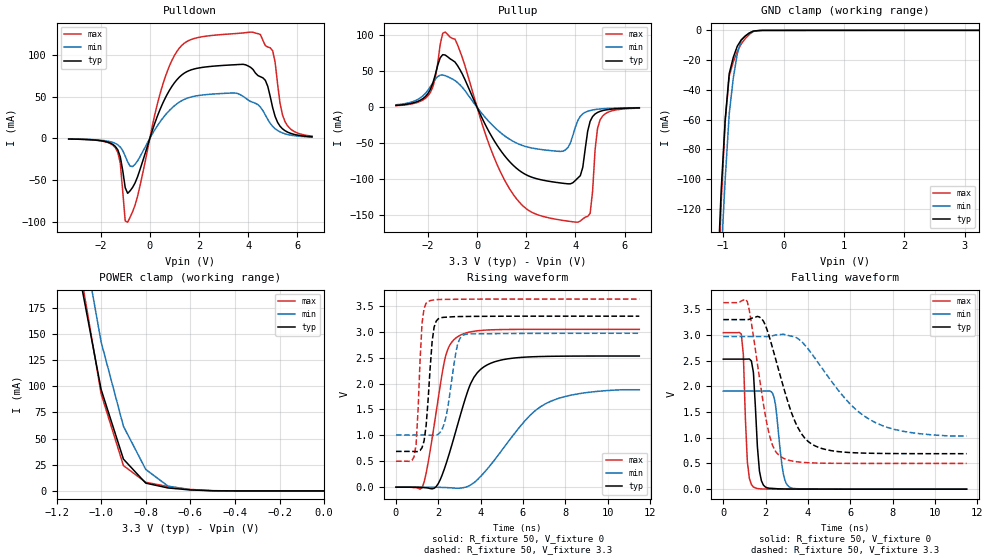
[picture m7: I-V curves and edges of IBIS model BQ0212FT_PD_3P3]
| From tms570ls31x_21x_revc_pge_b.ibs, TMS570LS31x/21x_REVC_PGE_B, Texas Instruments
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|   Model Cell BQ0212FT_PD_3P3
|BQ0212FT_PD_3P3
[Model]   BQ0212FT_PD_3P3
Model_type   I/O
Polarity   Non-Inverting
Enable   Active-Low
Vinl =  1.15
Vinh =  1.55
Cref =  15.0001pF
Rref =  101.0000M
Vref =  0V
Vmeas =  1.65
C_comp   1.2p   1.2p   1.2p
[Model Spec]
Vinl   1.15   1.02   1.28
Vinh   1.55   1.45   1.65
[Temperature Range]   25   155   -40
[Voltage Range]   3.3   2.97   3.63
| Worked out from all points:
|   slope of the pulldown table from 0 to 0.495 V, typ, clamps not added: 12.4 ohm
|   slope of the pullup table from 0 to 0.495 V, typ, clamps not added: 14.3 ohm
|   GND clamp passes 1 mA (typ) near -0.53 V on its own axis
|   POWER clamp passes 1 mA (typ) near -0.60 V on its own axis
|   rising waveform, R_fixture 50, V_fixture 0: 20-80 % time 1.15ns typ, 2.3ns min, 717ps max; typ from 0 V to 2.53 V
|   rising waveform, R_fixture 50, V_fixture 3.3: 20-80 % time 273ps typ, 440ps min, 219ps max; typ from 0.691 V to 3.3 V
|   falling waveform, R_fixture 50, V_fixture 0: 20-80 % time 219ps typ, 306ps min, 166ps max; typ from 2.53 V to 0 V
|   falling waveform, R_fixture 50, V_fixture 3.3: 20-80 % time 1.2ns typ, 2.39ns min, 725ps max; typ from 3.3 V to 0.691 V
[POWER_clamp]
|   voltage   I(typ)   I(min)   I(max)
-3.3V     3.99A      4.579A     4.788A
-1.1V     209.6mA    262.2mA    219.1mA
-1.067V   172.1mA    222.3mA    177mA
-1.033V   134.5mA    182.3mA    134.9mA
-1V       96.98mA    142.4mA    92.77mA
-900mV    30.41mA    61.81mA    24.23mA
-800mV    7.462mA    20.57mA    8.247mA
-700mV    2.848mA    4.595mA    4.228mA
-600mV    949.8uA    1.092mA    1.467mA
-500mV    155.7uA    238.9uA    226.8uA
0V        18.81uA    8.065uA    36.23uA
[Pulldown]
|   voltage   I(typ)   I(min)   I(max)
-3.3V     -649.5uA   -582.6uA   -652.5uA
-1.4V     -9.531mA   -5.889mA   -11.14mA
-1.2V     -22.05mA   -10.26mA   -29.81mA
-1V       -58.85mA   -20.91mA   -98.56mA
-900mV    -65.57mA   -28.22mA   -100.1mA
400mV     33.5mA     19.22mA    51.63mA
1.1V      70.16mA    41.36mA    104mA
4.1V      85.11mA    44.32mA    127.2mA
4.7V      69.58mA    28.18mA    111.1mA
5V        36.79mA    14.44mA    104.9mA
5.5V      9.351mA    5.597mA    20.3mA
6.6V      2.027mA    1.639mA    2.825mA
[Pullup]
|   voltage   I(typ)   I(min)   I(max)
-3.3V     2.63mA     3.499mA    2.212mA
-1.9V     24.96mA    28.62mA    20.66mA
-1.3V     72.58mA    44.01mA    104.4mA
-800mV    58.09mA    34.42mA    87.13mA
500mV     -34.83mA   -20.49mA   -52.76mA
1.5V      -81.5mA    -47.85mA   -122.3mA
3.5V      -105.5mA   -60.79mA   -157.1mA
4.1V      -98.13mA   -18.32mA   -159.5mA
4.6V      -19.34mA   -4.48mA    -147.3mA
4.8V      -9.331mA   -3.151mA   -59.41mA
5V        -5.707mA   -2.337mA   -17.88mA
6.6V      -794.7uA   -560.5uA   -1.138mA
[GND_clamp]
|   voltage   I(typ)   I(min)   I(max)
-3.3V     -3.259A    -2.879A    -4.965A
-1.1V     -172mA     -209.5mA   -194.3mA
-1.033V   -107.5mA   -151.2mA   -115.6mA
-966.7mV  -59.82mA   -100mA     -61.12mA
-900mV    -29.02mA   -56.02mA   -30.69mA
-833.3mV  -18.2mA    -32.15mA   -21.26mA
-766.7mV  -10.63mA   -15.71mA   -14.05mA
-700mV    -6.316mA   -6.699mA   -9.091mA
-566.7mV  -1.768mA   -1.723mA   -2.661mA
-500mV    -462.1uA   -565.3uA   -689.4uA
-366.7mV  -25.67uA   -48.26uA   -36.28uA
3.233V    18.8uA     10.51uA    36.2uA
[Ramp]
| variable   typ   min   max
dV/dt_f   1.604972/1.221205n   1.205115/2.49973n   1.9232/0.7363487n
dV/dt_r   1.538105/1.160119n   1.158114/2.384732n   1.850614/0.7248516n
R_load = 50
[Rising Waveform]
R_fixture = 50
V_fixture = 0
V_fixture_min = 0
V_fixture_max = 0
|   time   V(typ)   V(min)   V(max)
0s        -3.443uV   -1.451uV   -4.01uV
1.232ns   -5.491mV   -3.373uV   -11.5mV
1.516ns   -15.84mV   150.9uV    466.9mV
1.896ns   9.352mV    -960.2uV   1.442V
2.34ns    419.5mV    -6.879mV   2.522V
2.9ns     1.188V     -20.39mV   2.9V
3.684ns   2.121V     86.12mV    3.009V
4.472ns   2.391V     430.8mV    3.036V
7.08ns    2.524V     1.613V     3.046V
11.5ns    2.531V     1.88V      3.046V
[Rising Waveform]
R_fixture = 50
V_fixture = 3.3
V_fixture_min = 2.97
V_fixture_max = 3.63
|   time   V(typ)   V(min)   V(max)
0s        690.6mV    1.006V     501.3mV
852ps     689.3mV    1.006V     586.9mV
948ps     686.3mV    1.006V     818.8mV
1.232ns   763.6mV    1.006V     3.169V
1.516ns   1.676V     1.004V     3.584V
1.708ns   2.813V     998.6mV    3.607V
1.896ns   3.2V       1.003V     3.618V
2.34ns    3.28V      1.317V     3.624V
3.152ns   3.293V     2.93V      3.627V
11.5ns    3.3V       2.97V      3.63V
[Falling Waveform]
R_fixture = 50
V_fixture = 0
V_fixture_min = 0
V_fixture_max = 0
|   time   V(typ)   V(min)   V(max)
0s        2.531V     1.909V     3.046V
852ps     2.531V     1.909V     3.017V
1.136ns   2.531V     1.909V     540.4mV
1.424ns   2.271V     1.909V     42.46mV
1.708ns   353.8mV    1.909V     6.603mV
1.992ns   41.24mV    1.91V      3.131mV
2.4ns     12.71mV    1.783V     1.786mV
2.84ns    4.075mV    294mV      991.2uV
3.152ns   2.718mV    34.42mV    631.2uV
11.5ns    8.179uV    143.5uV    6.74uV
[Falling Waveform]
R_fixture = 50
V_fixture = 3.3
V_fixture_min = 2.97
V_fixture_max = 3.63
|   time   V(typ)   V(min)   V(max)
0s        3.3V       2.97V      3.63V
1.136ns   3.299V     2.97V      3.648V
1.708ns   3.35V      2.97V      2.172V
2.088ns   3.078V     2.969V     1.216V
2.716ns   2.172V     3.01V      633mV
3.528ns   1.196V     2.931V     530.7mV
4.472ns   817.8mV    2.467V     507.8mV
6.048ns   711.3mV    1.634V     501.8mV
7.284ns   696.3mV    1.276V     501.3mV
11.5ns    690.5mV    1.035V     501.3mV
